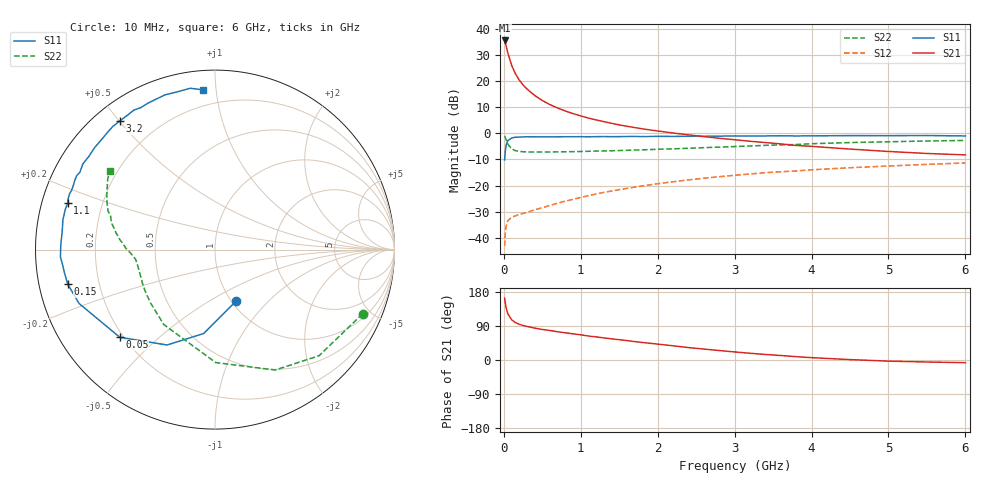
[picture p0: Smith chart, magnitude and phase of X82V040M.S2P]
! SIEMENS Small Signal Semiconductors
! BFP136W
! Si NPN RF Bipolar Junction Transistor in SOT343
! VCE = 2 V  IC = 40 mA
! Common Emitter S-Parameters:  September  1994
# GHz  S  MA  R  50
!  f  S11  S21  S12  S22
! GHz  MAG  ANG  MAG  ANG  MAG  ANG  MAG  ANG
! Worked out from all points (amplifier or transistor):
!   40 points, 10 MHz to 6 GHz, reference 50 ohm
!   highest |S21| = 35.6 dB at 10 MHz (marker M1)
!   |S21| within 3 dB of that: start of sweep to 37.15 MHz
!   unconditionally stable (mu >= 1): 621.7 MHz to 2.829 GHz
!   at 200 MHz: K = 0.51, MSG = 25.7 dB, |S12| = -31.0 dB
!   at 1.5 GHz: K = 1.13, MAG = 10.2 dB, |S12| = -21.6 dB
!   at 6 GHz: K = 0.98, MSG = 1.5 dB, |S12| = -11.3 dB
!   S11 on the Smith chart (normalised r, x): 10 MHz: 1.05, -0.67; 50 MHz: 0.19, -0.38; 150 MHz: 0.09, -0.11; 1.1 GHz: 0.08, +0.15; 3.2 GHz: 0.07, +0.50; 6 GHz: 0.11, +0.92
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0.01  0.3095 -67.4  60.28 163.5  0.0069 73.4  0.8972 -23.5
0.02  0.4718 -97.7  53.82 149.0  0.0128 60.8  0.8278 -45.6
0.03  0.5949 -116.7  47.33 137.8  0.0166 52.1  0.7502 -63.4
0.05  0.7211 -137.4  35.43 122.9  0.0209 38.8  0.6296 -89.6
0.1  0.8149 -158.4  20.32 106.3  0.0248 30.2  0.5058 -124.3
0.15  0.8429 -166.8  13.95 98.8  0.0262 29.6  0.4662 -140.5
0.2  0.8489 -171.5  10.49 94.3  0.0281 31.7  0.4522 -149.7
0.25  0.8548 -174.9  8.475 91.0  0.0293 33.1  0.4453 -155.4
0.3  0.8622 -177.3  7.089 88.5  0.0306 36.2  0.4407 -159.3
0.4  0.8597 178.6  5.341 84.2  0.0343 40.5  0.4391 -164.3
0.5  0.8577 175.6  4.261 80.6  0.0376 43.9  0.4394 -167.5
0.6  0.8571 173.4  3.55 77.8  0.0417 47.3  0.4407 -169.5
0.7  0.8603 170.8  3.062 74.5  0.046 50.0  0.442 -170.8
0.9  0.8629 167.1  2.394 69.0  0.0545 53.4  0.4465 -173.2
1.1  0.8602 162.5  1.959 63.2  0.064 55.1  0.4538 -174.6
1.5  0.8661 155.9  1.453 53.6  0.0835 56.7  0.4688 -177.3
1.8  0.8675 150.2  1.224 46.3  0.0984 56.0  0.4833 -179.5
2.2  0.8739 143.5  1.016 37.5  0.1182 54.2  0.5054 177.6
3.2  0.8916 126.4  0.706 17.8  0.1666 46.4  0.5729 168.3
4.5  0.9061 108.0  0.5 1.1  0.2196 34.4  0.6666 154.9
5.5  0.9094 98.7  0.412 -5.3  0.2545 26.3  0.7152 146.7
6  0.8927 94.4  0.387 -7.0  0.2712 21.8  0.7325 143.2
